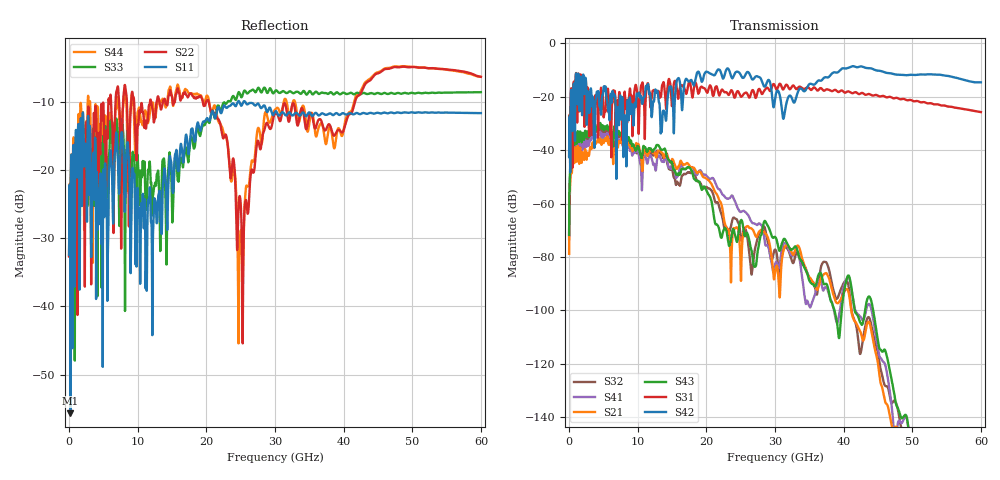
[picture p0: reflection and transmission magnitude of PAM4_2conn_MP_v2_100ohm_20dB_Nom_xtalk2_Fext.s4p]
! Info: Touchstone file created by Circ.  Input file=FAB50GbE_2conn_Midplane_Examax_Topo2_v2_100ohm_20dB_Nom.circ
# Hz S RI R 50
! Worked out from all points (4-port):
!   6000 points, 10 MHz to 60 GHz, reference 50 ohm
!   strongest paths, dB at 10 MHz, 15.01 GHz, 30.01 GHz, 45.01 GHz, 60 GHz:
!     S42: -42.6, -18.4, -20.8, -10.2, -14.6
!     S31: -42.1, -23.2, -16.0, -19.6, -25.7
!     S43: -71.7, -44.6, -72.5, -111.5, -157.2
!     S21: -78.8, -43.3, -86.0, -119.9, -163.0
!     S41: -71.6, -44.8, -82.8, -114.2, -166.9
!     S32: -73.3, -46.8, -77.2, -116.0, -160.2
!   lowest |S11| = -55.7 dB at 190 MHz (marker M1), VSWR 1.00, Z = 49.9 - j0.154 ohm
!   |S11| at or under -10 dB: start of sweep to 24.61 GHz; 24.79 GHz to 25.43 GHz (645.3 MHz wide, 2.57 % of centre); 25.63 GHz to end of sweep
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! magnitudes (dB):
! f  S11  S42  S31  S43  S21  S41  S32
! 10 MHz  -32.4  -42.6  -42.1  -71.7  -78.8  -71.6  -73.3
! 190 MHz  -55.7  -29.7  -28.7  -44.5  -49.4  -46.4  -46.3
! 7.5 GHz  -17.1  -20.0  -22.3  -34.0  -37.1  -36.7  -35.1
! 20.15 GHz  -12.4  -10.7  -18.5  -55.8  -50.9  -50.0  -54.0
! 24.86 GHz  -10.2  -11.1  -19.1  -67.6  -74.7  -62.9  -69.1
! 27.01 GHz  -10.5  -12.8  -18.9  -83.6  -71.1  -67.4  -78.1
! 60 GHz  -11.7  -14.6  -25.7  -157.2  -163.0  -166.9  -160.2
